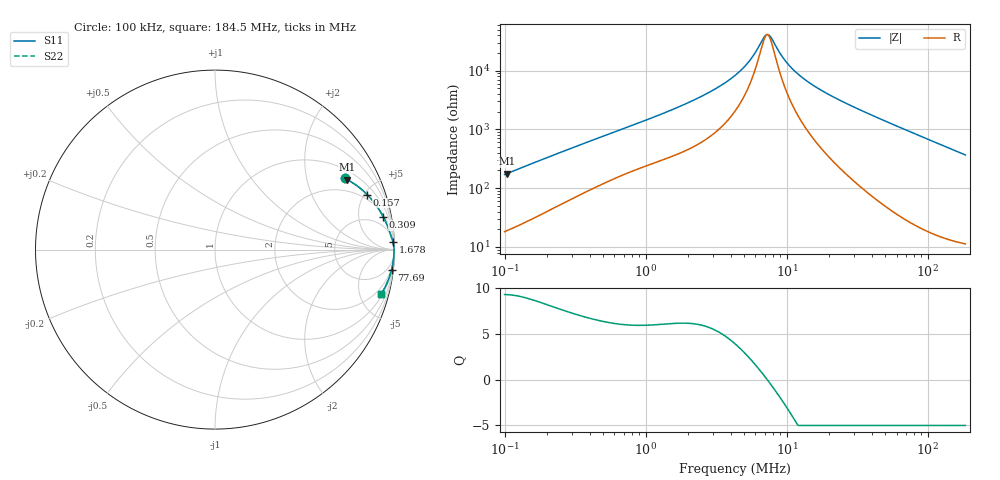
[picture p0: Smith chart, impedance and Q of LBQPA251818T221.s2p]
! LBQPA251818T221  S-PARAMETER MODEL  ( General Type )
! Model Generated by TAIYO YUDEN Corporation (http://www.ty-top.com)
! Version 1.0
! TAIYO YUDEN Control No. 191025NI43SB-FBB
! Copyright(c) 2019 TAIYO YUDEN CO.,LTD. All Rights Reserved.
! Product Description (link to TY-COMPAS)
! https://ds.yuden.co.jp/TYCOMPAS/or/detail?pn=LBQPA251818T221K&u=M
! Products Name : Inductors
! Characteristics :
!  Inductance : 220 uH , SRF(min) : 5.5 MHz , DC Resistance(max) : 10.92 Ohm
!  Rated Current : Saturation :115 mA , Temp Rise : 80 mA (20 degC)
!  Case Size : 2.5 x 1.8 / 0.098 x 0.071 [mm/inch] , Thickness : 1.8 / 0.071 [mm/inch]
!  (Conditions: Temperature = 25 degC , DC Bias Current/Voltage = 0A / 0V)
! External Node Assignments :
!  1  o---GGG---o  2
! GND o---------o GND
! Frequency Range : 0.1MHz  -  184.468258MHz  [ 402 STEP ]
# MHz S RI R 50
! Freq[MHz].  S11 Real  S11 Imag  S21 Real  S21 Imag  S12 Real  S12 Imag  S22 Real  S22 Imag
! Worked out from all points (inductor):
!   401 points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, 100 kHz to 184.5 MHz, reference 50 ohm
!   read as one part in series: L = 268 uH near 103.8 kHz
!   highest Q = 9.29 at 103.8 kHz (marker M1), where L = 270 uH
!   self-resonance near 7.271 MHz
!   S11 on the Smith chart (normalised r, x): 100 kHz: 1.37, +3.40; 157 kHz: 1.60, +5.24; 308.9 kHz: 2, +10; 1.678 MHz: 9, +47; 77.69 MHz: 1, -18; 184.5 MHz: 1.23, -7.34
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0.1  0.7238 0.3966  0.2762 -0.3966  0.2762 -0.3966  0.7238 0.3966
0.103832  0.7366 0.3899  0.2634 -0.3899  0.2634 -0.3899  0.7366 0.3899
0.15702  0.8479 0.3064  0.1521 -0.3064  0.1521 -0.3064  0.8479 0.3064
0.30895  0.9376 0.1823  0.0624 -0.1823  0.0624 -0.1823  0.9376 0.1823
0.352405  0.9469 0.1634  0.0531 -0.1634  0.0531 -0.1634  0.9469 0.1634
1.241892  0.9877 0.0551  0.0123 -0.0551  0.0123 -0.0551  0.9877 0.0551
1.677724  0.9916 0.0412  0.00845 -0.0412  0.00845 -0.0412  0.9916 0.0412
2.948932  0.9957 0.0215  0.00434 -0.0215  0.00434 -0.0215  0.9957 0.0215
4.294977  0.9969 0.0117  0.00312 -0.0117  0.00312 -0.0117  0.9969 0.0117
5.381935  0.9973 0.00649  0.00271 -0.00649  0.00271 -0.00649  0.9973 0.00649
5.912382  0.9974 0.00443  0.0026 -0.00443  0.0026 -0.00443  0.9974 0.00443
6.871965  0.9975 0.0012  0.00246 -0.0012  0.00246 -0.0012  0.9975 0.0012
7.270685  0.9976 3.92e-07  0.00242 -3.92e-07  0.00242 -3.92e-07  0.9976 3.92e-07
7.69254  0.9976 -0.0012  0.00239 0.0012  0.00239 0.0012  0.9976 -0.0012
9.110726  0.9977 -0.00486  0.00234 0.00486  0.00234 0.00486  0.9977 -0.00486
10.39218  0.9977 -0.00779  0.00233 0.00779  0.00233 0.00779  0.9977 -0.00779
12.30807  0.9976 -0.0118  0.00237 0.0118  0.00237 0.0118  0.9976 -0.0118
15.13571  0.9975 -0.0171  0.0025 0.0171  0.0025 0.0171  0.9975 -0.0171
24.67673  0.9967 -0.0331  0.00334 0.0331  0.00334 0.0331  0.9967 -0.0331
53.33896  0.9915 -0.0765  0.00853 0.0765  0.00853 0.0765  0.9915 -0.0765
77.68562  0.9841 -0.1117  0.0159 0.1117  0.0159 0.1117  0.9841 -0.1117
184.4683  0.9244 -0.2495  0.0756 0.2495  0.0756 0.2495  0.9244 -0.2495
